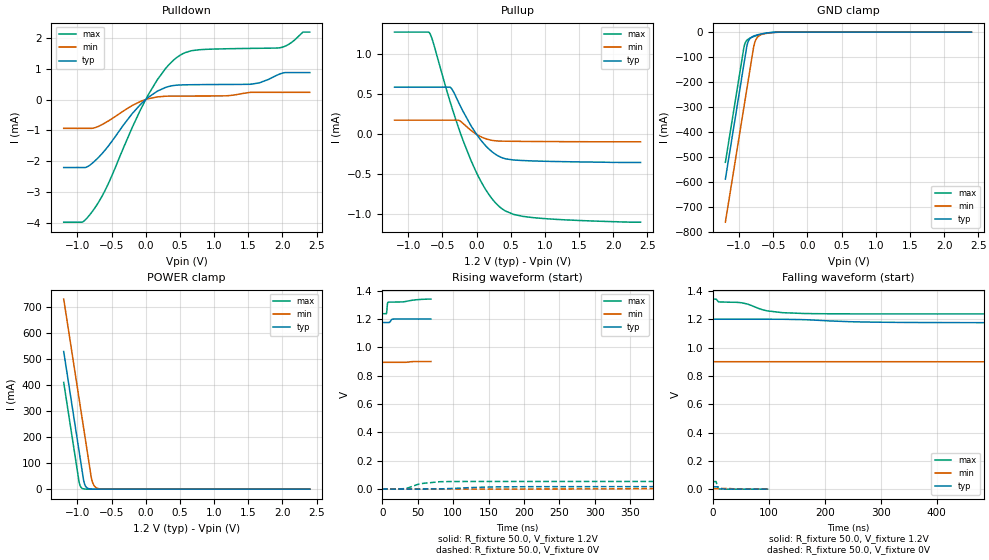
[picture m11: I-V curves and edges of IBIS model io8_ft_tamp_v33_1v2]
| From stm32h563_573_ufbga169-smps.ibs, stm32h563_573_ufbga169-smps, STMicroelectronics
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[Model]   io8_ft_tamp_v33_1v2
Model_type I/O
Polarity   Non-Inverting
Enable   Active-Low
| CAP_THRESHOLD on pad IOFT is "UDTCAPC" :
| Rising=20.0% of vddiom   Falling=80.0% of vddiom
| C_comp min and max val. don't necessarily correlate with the min and max pvt
| but are the smallest and greatest pad capacitance found.
| var   typ   min   max
C_comp   6.62990pF  6.52955pF  6.96695pF
|C_comp_pullup   3.55120pF  3.69070pF  4.15080pF
|C_comp_pulldown   3.07870pF  2.83885pF  2.81615pF
Vinl = 450.0mV
Vinh = 660.0mV
Vmeas = 600.0mV   | Reference voltage for timing measurements
Cref  = 50.0pF   | Timing specification test load capacitance value
Rref  = 1.0MOhm   | Timing specification test load resistance value
Vref  = 660.0mV   | Timing specification test load voltage
[Model Spec]
| TIME_THRESHOLD on pin ZIV33SW is "CMOS" :
| Rising=40.0% of VDDV33SW   Falling=60.0% of VDDV33SW
Vinl 443.80000mV 340.80000mV 585.80000mV
Vinh 727.20000mV 529.20000mV 933.20000mV
| variable   typ   min   max
[Temperature Range] 25.0 125.0 -40.0
| variable   typ   min   max
[Voltage Range] 1.2V 900.0mV 1.32V
| variable   typ   min   max
[POWER Clamp Reference] 1.2V 900.0mV 1.32V
| variable   typ   min   max
[GND Clamp Reference] 0V 0V 0V
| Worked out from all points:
|   slope of the pulldown table from 0 to 0.18 V, typ, clamps not added: 640 ohm
|   slope of the pullup table from 0 to 0.18 V, typ, clamps not added: 985 ohm
|   GND clamp passes 1 mA (typ) near -0.49 V on its own axis
|   POWER clamp passes 1 mA (typ) near -0.82 V on its own axis
[POWER Clamp]
-1.2V     528.6mA    730.2mA    409.9mA
-970mV    137.6mA    339.2mA    21.83mA
-950mV    103.6mA    305.2mA    8.066mA
-910mV    35.64mA    237.2mA    1.102mA
-890mV    16.36mA    203.2mA    407.1uA
-850mV    3.449mA    135.2mA    55.6uA
-800mV    492.6uA    50.22mA    4.616uA
-790mV    333.8uA    37.52mA    2.807uA
-760mV    103.8uA    15.65mA    630.8nA
-730mV    32.3uA     6.528mA    141.9nA
-580mV    94.87nA    82.18uA    221.4pA
2.4V      0A         0A         0A
[GND Clamp]
-1.2V     -589.6mA   -762.3mA   -522.3mA
-930mV    -130.6mA   -303.3mA   -63.3mA
-920mV    -113.6mA   -286.3mA   -51.27mA
-890mV    -62.61mA   -235.3mA   -34.26mA
-870mV    -40.55mA   -201.3mA   -29.23mA
-840mV    -25.72mA   -150.3mA   -24.37mA
-780mV    -15.34mA   -52.09mA   -17.43mA
-750mV    -12.56mA   -28.41mA   -14.57mA
-710mV    -9.614mA   -15.23mA   -11.15mA
-590mV    -3.598mA   -4.725mA   -3.7mA
-360mV    -55.33uA   -263.2uA   -15.15uA
2.4V      4.717nA    981.3nA    269.8pA
| variable   typ   min   max
[Pullup Reference] 1.2V 900.0mV 1.32V
| variable   typ   min   max
[Pulldown Reference] 0V 0V 0V
[Pullup]
-1.2V     589.6uA    177.1uA    1.277mA
-700mV    589.6uA    177.1uA    1.277mA
-680mV    589.6uA    177.1uA    1.255mA
-630mV    589.6uA    177.1uA    1.135mA
-380mV    584.7uA    177.1uA    387.9uA
-250mV    376.7uA    171.5uA    48.5uA
-80mV     105.5uA    47.7uA     -329.9uA
140mV     -148.8uA   -56.28uA   -698.9uA
360mV     -287.4uA   -84.53uA   -921.6uA
540mV     -320.3uA   -86.94uA   -999.2uA
790mV     -331.1uA   -88.82uA   -1.037mA
2.4V      -351uA     -93uA      -1.097mA
[Pulldown]
-1.2V     -2.205mA   -936uA     -3.978mA
-930mV    -2.205mA   -936uA     -3.978mA
-740mV    -1.984mA   -912uA     -3.502mA
-560mV    -1.545mA   -713.6uA   -2.789mA
40mV      74.37uA    26.48uA    163.8uA
290mV     391.1uA    106.7uA    1.004mA
450mV     464.1uA    111.5uA    1.354mA
670mV     479.4uA    113uA      1.582mA
1.53V     494.1uA    231.8uA    1.657mA
1.97V     833.4uA    231.8uA    1.682mA
2.3V      872.5uA    231.8uA    2.186mA
2.4V      872.5uA    231.8uA    2.186mA
[Ramp]
dV/dt_r 10.18837mV/50.29263ns 2.6744mV/147.58995ns 31.996mV/21.07202ns
dV/dt_f 14.63972mV/94.15205ns 3.40945mV/266.09455ns 62.6599mV/86.25178ns
R_load = 50.0
| Removed startup time: 0s 0s 0s  .
| Removed end time: 68.75ns.
[Rising Waveform]
R_fixture   = 50.0
V_fixture   = 1.2V
V_fixture_min = 900.0mV
V_fixture_max = 1.32V
0s        1.176V     894.3mV    1.238V
5.75ns    1.176V     894.3mV    1.238V
6.4ns     1.176V     894.3mV    1.254V
7.45ns    1.176V     894.3mV    1.31V
8.4ns     1.176V     894.3mV    1.319V
9.85ns    1.175V     894.3mV    1.32V
12.75ns   1.194V     894.3mV    1.32V
15.45ns   1.2V       894.3mV    1.32V
29.5ns    1.2V       894.3mV    1.322V
68.75ns   1.2V       900mV      1.341V
| Removed startup time: 0s 0s 0s  .
| Removed end time: 1.99875us.
[Falling Waveform]
R_fixture   = 50.0
V_fixture   = 1.2V
V_fixture_min = 900.0mV
V_fixture_max = 1.32V
0s        1.2V       900mV      1.342V
5.4ns     1.2V       900mV      1.342V
10.8ns    1.2V       900mV      1.322V
51.35ns   1.2V       900mV      1.316V
96.6ns    1.2V       900mV      1.259V
125.2ns   1.2V       900mV      1.246V
180ns     1.194V     900mV      1.239V
253.1ns   1.182V     900mV      1.238V
407.9ns   1.176V     899.9mV    1.238V
1.999us   1.176V     894.3mV    1.238V
| Removed startup time: 0s 0s 0s  .
| Removed end time: 1.9987us.
[Rising Waveform]
R_fixture   = 50.0
V_fixture   = 0V
V_fixture_min = 0V
V_fixture_max = 0V
0s        76.86nV    1.65uV     79.77nV
31.1ns    -18.91uV   -9.669uV   2.514mV
36.5ns    -18.91uV   -59.88uV   8.399mV
55ns      16.66uV    -10.51uV   38.69mV
81.6ns    1.041mV    -2.484uV   51.73mV
98.1ns    3.976mV    -2.232uV   52.89mV
163.2ns   15.18mV    16.21uV    53.28mV
244.8ns   16.86mV    234.8uV    53.3mV
571.1ns   16.96mV    4.288mV    53.32mV
1.999us   16.98mV    4.459mV    53.33mV
| Removed startup time: 0s 0s 0s  .
| Removed end time: 98.75ns.
[Falling Waveform]
R_fixture   = 50.0
V_fixture   = 0V
V_fixture_min = 0V
V_fixture_max = 0V
0s        16.99mV    4.473mV    53.33mV
5.3ns     16.99mV    4.473mV    53.57mV
7.75ns    17mV       4.473mV    20.42mV
8.8ns     16.92mV    4.473mV    9.656mV
9.95ns    14.09mV    4.473mV    4.317mV
12.1ns    8.742mV    4.473mV    882.3uV
16.15ns   2.326mV    4.473mV    170.2uV
24.2ns    154.7uV    4.471mV    27.86uV
52.4ns    6.19uV     441.6uV    23.35uV
98.75ns   4.959uV    12.26uV    9.525uV
